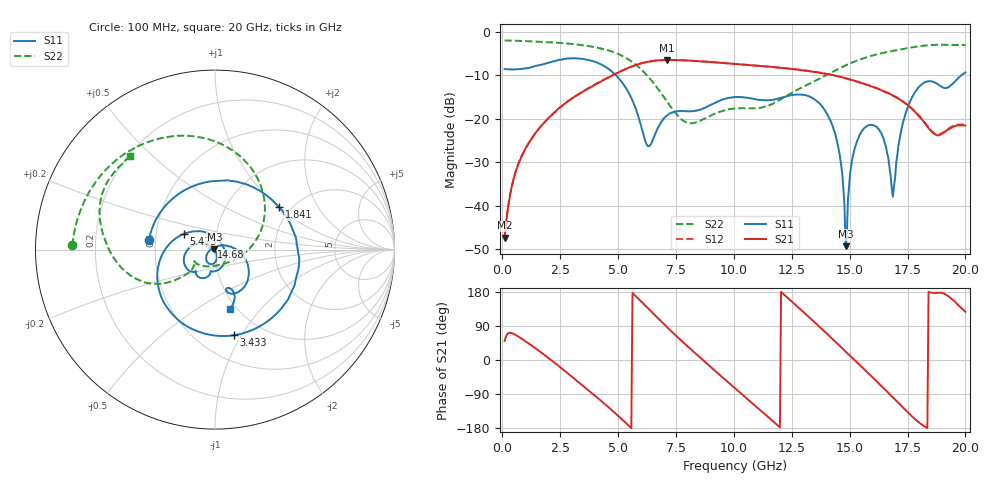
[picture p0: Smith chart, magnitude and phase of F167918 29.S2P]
!  2-Port S-parameters saved by WinCal
! VAR MeasName=S-Parameters (CALIBRATED_DATA) read from VNA (N5242A)
! VAR MeasDate=2016-11-22 10:26:08
! VAR NAME=F167918 29
! VAR FILENAME=F167918 29.S2P
! VAR DATE=2016-11-22 10:26:08
! VAR PHYS_PORTS=1,2
# Hz S DB R 50
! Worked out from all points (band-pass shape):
!   401 points, 100 MHz to 20 GHz, reference 50 ohm
!   highest |S21| = -6.48 dB at 7.115 GHz (marker M1); lowest = -47.4 dB at 100 MHz (marker M2)
!   |S21| within 3 dB of the highest: 4.972 GHz to 13.78 GHz (8.811 GHz wide, 94 % of centre)
!   lowest |S11| = -49.4 dB at 14.83 GHz (marker M3), VSWR 1.01, Z = 49.7 + j0.0664 ohm
!   |S11| at or under -10 dB: 4.903 GHz to 19.83 GHz (14.93 GHz wide, 121 % of centre)
!   |S22| runs from -21.1 to -2.0 dB; largest |S21 - S12| = 0.0041
!   S11 on the Smith chart (normalised r, x): 100 MHz: 0.46, +0.06; 1.841 GHz: 1.74, +1.01; 3.433 GHz: 0.74, -0.93; 5.473 GHz: 0.69, +0.13; 14.68 GHz: 0.96, +0.03; 20 GHz: 0.93, -0.70
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1e8  -8.59 171.3  -47.40 50.6  -47.35 50.2  -2.00 178.3
6.97e8  -8.62 122.5  -30.41 61.8  -30.37 61.5  -2.09 168.8
1.84125e9  -7.38 33.6  -20.73 12.2  -20.72 12.1  -2.34 150.4
3.43325e9  -6.22 -77.6  -13.93 -65.6  -13.87 -65.4  -3.07 120.5
5.473e9  -14.18 153.4  -8.25 -173.9  -8.24 -174.3  -6.45 61.9
6.269e9  -26.24 45.3  -6.92 137.8  -6.94 137.6  -10.15 29.7
6.7665e9  -21.68 -48.7  -6.56 107.3  -6.57 107.3  -13.46 7.4
7.11475e9  -19.24 -74.3  -6.48 86.5  -6.50 86.6  -16.06 -9.8
8.5575e9  -17.91 -101.1  -6.80 5.4  -6.78 5.4  -20.47 -102.1
1.005e10  -15.02 -118.6  -7.40 -74.4  -7.40 -74.3  -17.69 -146.6
1.179125e10  -15.53 -132.1  -8.18 -166.9  -8.15 -166.9  -16.26 -141.2
1.338325e10  -15.25 -169.0  -9.14 105.4  -9.13 105.5  -11.64 -141.7
1.4229e10  -21.18 156.5  -9.93 57.2  -9.93 57.3  -9.32 -146.8
1.467675e10  -32.41 138.2  -10.46 31.1  -10.47 31.2  -8.15 -151.1
1.4826e10  -49.35 168.7  -10.73 22.2  -10.70 22.5  -7.74 -152.7
1.517425e10  -27.92 -74.4  -11.20 2.0  -11.21 2.3  -6.96 -157.4
1.5622e10  -22.22 -94.5  -11.97 -23.9  -11.98 -23.7  -6.06 -163.7
1.67165e10  -31.05 -174.0  -14.22 -89.3  -14.25 -88.8  -4.57 179.8
1.69155e10  -35.61 80.9  -14.84 -101.2  -14.76 -100.9  -4.34 176.8
1.73135e10  -20.70 10.1  -16.11 -125.9  -16.06 -125.2  -3.96 171.3
1.796025e10  -12.92 -33.6  -19.23 -163.1  -19.07 -162.4  -3.36 161.6
2e10  -9.35 -75.9  -21.55 127.0  -21.35 127.3  -3.05 132.3
